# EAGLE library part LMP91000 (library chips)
IC TI AFE for Gas Sensing
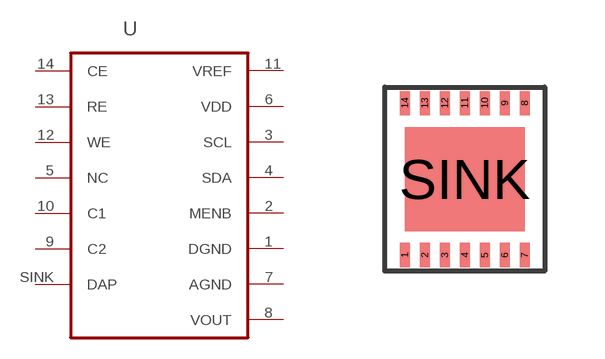
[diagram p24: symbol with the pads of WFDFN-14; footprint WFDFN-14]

Designator prefix -

## LMP91000 (DIGIKEY: LMP91000SDE/NOPBCT-ND)  [WFDFN-14]
1  DGND  pas
2  MENB  pas
3  SCL
4  SDA  pas
5  NC  pas
6  VDD  pwr
7  AGND  pas
8  VOUT  pas
9  C2  pas
10  C1  pas
11  VREF  pwr
12  WE
13  RE
14  CE
SINK  DAP  pas

## Footprint WFDFN-14 (pad centres in mm)
smd 0.25 x 0.6: 1 -1.5,-1.9; 2 -1,-1.9; 3 -0.5,-1.9; 4 0,-1.9; 5 0.5,-1.9; 6 1,-1.9; 7 1.5,-1.9; 8 1.5,1.9; 9 1,1.9; 10 0.5,1.9; 11 0,1.9; 12 -0.5,1.9; 13 -1,1.9; 14 -1.5,1.9
smd 3 x 2.6: SINK 0,0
